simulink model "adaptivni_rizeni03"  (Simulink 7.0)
settings: Solver=ode45  SolverMode=SingleTasking  StartTime=0.0  StopTime=100  RelTol=1e-3  AbsTol=1e-6
PostLoadFcn:
  | ex12par
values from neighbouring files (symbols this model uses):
  a = 1    [example_3_5_2_podklad.m]
  am = 2    [example_3_5_2_podklad.m]
  b = 0.5    [example_3_5_2_podklad.m]
  bm = 2    [example_3_5_2_podklad.m]
  gamma = 1    [example_3_5_2_podklad.m]
libraries: simulink x1

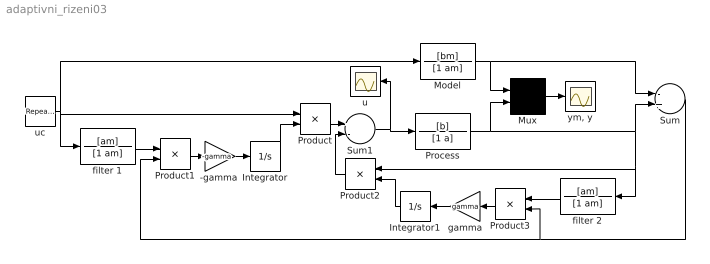
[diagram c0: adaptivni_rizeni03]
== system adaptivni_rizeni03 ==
  "-gamma " : Gain  Gain=-gamma  ParameterDataType=sfix(16)  ParameterScaling=2^0  OutDataType=sfix(16)  OutScaling=2^0
  Integrator : Integrator
  Integrator1 : Integrator  Orientation=left
  Model : TransferFcn  Numerator=[bm]  Denominator=[1 am]
  Mux : Mux  Inputs=2
  Process : TransferFcn  Numerator=[b]  Denominator=[1 a]
  Product : Product  OutDataType=sfix(16)  OutScaling=2^0
  Product1 : Product  OutDataType=sfix(16)  OutScaling=2^0
  Product2 : Product  Orientation=left  OutDataType=sfix(16)  OutScaling=2^0
  Product3 : Product  Orientation=left  OutDataType=sfix(16)  OutScaling=2^0
  Sum : Sum  Inputs=-+  OutDataType=sfix(16)  OutScaling=2^0
  Sum1 : Sum  Inputs=+-  OutDataType=sfix(16)  OutScaling=2^0
  filter 1 : TransferFcn  Numerator=[am]  Denominator=[1 am]
  filter 2 : TransferFcn  Orientation=left  Numerator=[am]  Denominator=[1 am]
  gamma : Gain  Orientation=left  Gain=gamma  ParameterDataType=sfix(16)  ParameterScaling=2^0  OutDataType=sfix(16)  OutScaling=2^0
  u : Scope
  uc : simulink/Sources/Repeating Sequence  SystemSampleTime=-1  rep_seq_t=[0 10 10 20]  rep_seq_y=[1 1 -1 -1]
  "ym, y" : Scope
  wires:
  Product/1 -> Sum1/1
  "-gamma "/1 -> Integrator/1
  Product1/1 -> "-gamma "/1
  filter 1/1 -> Product1/1
  uc/1 -> Product/1, Model/1, filter 1/1
  filter 2/1 -> Product3/1
  gamma/1 -> Integrator1/1
  Product3/1 -> gamma/1
  Sum/1 -> Product1/2, Product3/2
  Process/1 -> Sum/2, Product2/1, filter 2/1, Mux/2
  Model/1 -> Sum/1, Mux/1
  Mux/1 -> "ym, y"/1
  Sum1/1 -> Process/1, u/1
  Integrator/1 -> Product/2
  Product2/1 -> Sum1/2
  Integrator1/1 -> Product2/2
